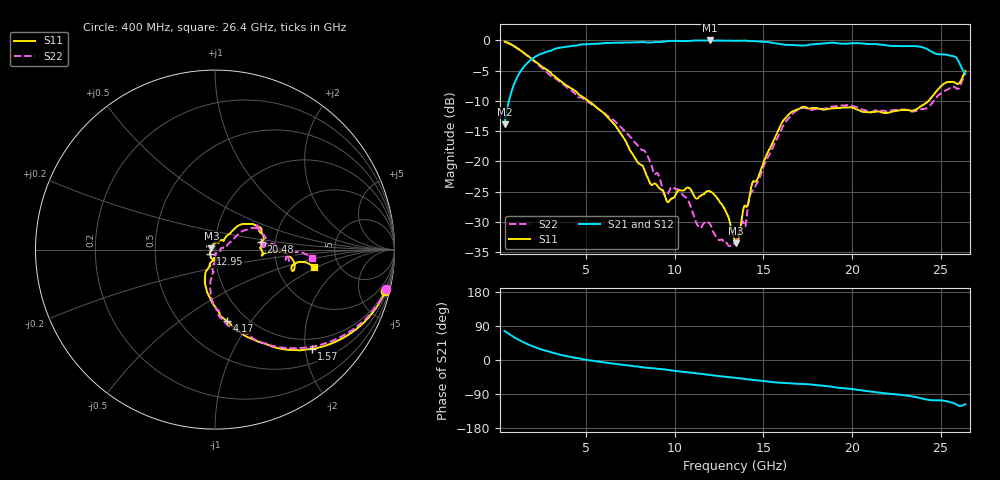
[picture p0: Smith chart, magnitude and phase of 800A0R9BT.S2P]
!  American Technical Ceramics  Date:  12/17/08
!  One Norden Lane
!  Huntington Station,  NY.  11746-2102
!  Tel:  (631) 622-4700  Fax:  (631) 622-4748
!  Part Number  800A0R9BT
!  Description: Broardband capacitor  Mounting Orientation: Vertical
!  Application:
# GHZ S DB R 50
! Freq  |S11|  S11 Ph  |S21|  S21 Ph  |S12|  S12 Ph  |S22|  S22 Ph
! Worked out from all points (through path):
!   401 points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, 400 MHz to 26.4 GHz, reference 50 ohm
!   highest |S21| = 0.00 dB at 11.97 GHz (marker M1); lowest = -13.8 dB at 400 MHz (marker M2)
!   lowest |S11| = -33.5 dB at 13.46 GHz (marker M3), VSWR 1.04, Z = 48 + j0.645 ohm
!   |S11| at or under -10 dB: 5.126 GHz to 24.32 GHz (19.19 GHz wide, 130 % of centre)
!   |S22| runs from -34.0 to -0.2 dB; largest |S21 - S12| = 0.0025
!   S11 on the Smith chart (normalised r, x): 400 MHz: 0.80, -8.23; 1.57 GHz: 0.78, -2.13; 4.17 GHz: 0.81, -0.77; 12.95 GHz: 0.95, -0.05; 20.48 GHz: 1.68, +0.15; 26.4 GHz: 3.26, -0.93
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0.4  -0.20 -13.7  -13.84 76.4  -13.85 76.4  -0.19 -12.9
0.92  -0.91 -29.8  -7.35 60.6  -7.35 60.5  -0.92 -28.4
1.57  -2.25 -45.7  -4.07 44.4  -4.07 44.4  -2.27 -44.5
2.675  -4.63 -62.8  -1.98 25.3  -1.98 25.3  -4.96 -64.6
4.17  -7.93 -80.6  -0.92 7.7  -0.92 7.7  -8.27 -84.7
4.755  -9.24 -86.8  -0.66 2.6  -0.67 2.6  -9.47 -88.3
7.29  -16.99 -112.2  -0.35 -14.0  -0.35 -14.0  -15.32 -97.7
9.11  -24.36 -98.4  -0.28 -23.5  -0.28 -23.4  -22.39 -91.2
9.63  -26.74 -89.2  -0.09 -26.2  -0.09 -26.1  -25.28 -67.7
11.385  -25.78 -93.4  -0.01 -36.3  -0.01 -36.2  -30.98 -87.1
11.97  -24.88 -103.1  0.00 -39.8  -0.01 -39.8  -30.26 -91.9
12.945  -28.70 -136.8  -0.02 -44.8  -0.02 -44.8  -33.57 -69.6
13.4  -33.17 173.2  -0.06 -47.0  -0.06 -47.0  -33.39 -35.6
13.465  -33.53 161.4  -0.06 -47.3  -0.06 -47.3  -33.08 -29.9
14.375  -23.55 52.6  -0.11 -52.0  -0.10 -52.0  -24.91 9.1
16.065  -13.47 42.4  -0.66 -60.3  -0.66 -60.3  -14.40 33.7
17.755  -11.18 22.0  -0.64 -65.1  -0.63 -65.1  -11.47 27.5
20.485  -11.68 9.3  -0.47 -80.0  -0.46 -80.0  -11.32 6.5
22.11  -11.91 1.4  -0.87 -89.1  -0.87 -89.1  -11.59 8.3
23.93  -10.78 -4.0  -1.09 -101.3  -1.08 -101.4  -11.37 2.6
25.945  -7.18 -13.9  -3.06 -118.8  -3.06 -118.7  -8.01 -8.1
26.4  -5.03 -10.1  -5.45 -116.6  -5.44 -116.8  -5.34 -4.9
